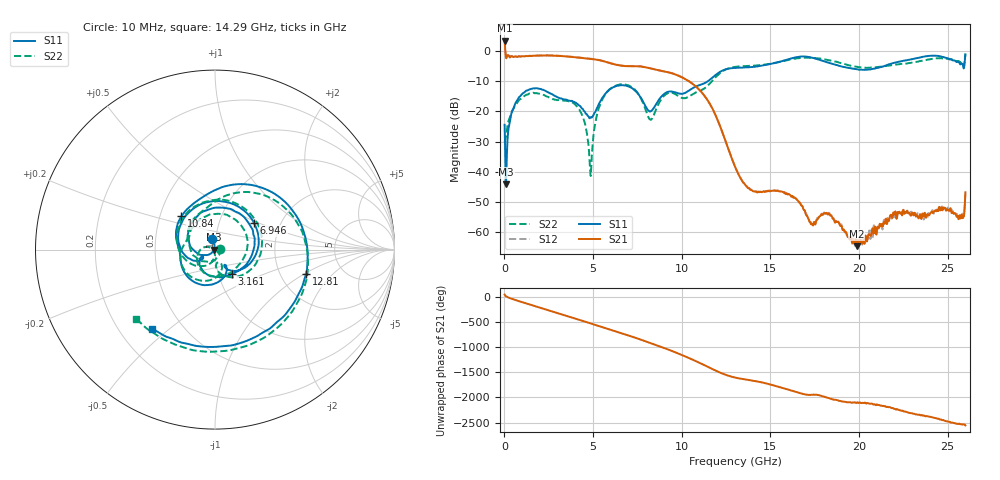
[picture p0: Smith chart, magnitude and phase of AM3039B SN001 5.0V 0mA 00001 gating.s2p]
!Agilent Technologies,E8364B,MY43040894,A.07.50.67
!Agilent E8364B: A.07.50.67
!Date: Tuesday, June 28, 2016 08:03:35
!Correction: S11(Full 2 Port(1,2))
!S21(Full 2 Port(1,2))
!S12(Full 2 Port(1,2))
!S22(Full 2 Port(1,2))
!S2P File: Measurements: S11, S21, S12, S22:
# Hz S  dB  R 50
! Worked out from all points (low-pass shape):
!   1601 points, 10 MHz to 26 GHz, reference 50 ohm
!   highest |S21| = 3.53 dB at 10 MHz (marker M1); lowest = -64.8 dB at 19.88 GHz (marker M2)
!   |S21| within 3 dB of the highest: start of sweep to 44.86 MHz
!   lowest |S11| = -44.2 dB at 91.22 MHz (marker M3), VSWR 1.01, Z = 49.4 + j0.00893 ohm
!   |S11| at or under -10 dB: start of sweep to 11.46 GHz
!   |S22| runs from -41.4 to -0.7 dB; largest |S21 - S12| = 0.024
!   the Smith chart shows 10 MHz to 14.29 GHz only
!   S11 on the Smith chart (normalised r, x): 10 MHz: 0.96, +0.11; 3.161 GHz: 1.16, -0.32; 6.946 GHz: 1.46, +0.47; 10.84 GHz: 0.64, +0.26; 12.81 GHz: 2.78, -1.03; 14.29 GHz: 0.34, -0.44
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1e7  -24.43 104.9  3.53 40.5  3.59 41.3  -30.33 10.6
9.121875e7  -44.21 179.2  -2.20 4.6  -2.10 4.6  -28.23 -60.6
7.572125e8  -16.00 158.6  -1.76 -84.1  -1.71 -83.8  -16.80 171.7
1.650619e9  -12.32 66.5  -1.50 179.4  -1.45 179.6  -13.79 70.0
3.161288e9  -15.71 -55.8  -1.57 15.8  -1.52 16.1  -16.23 -57.9
4.347081e9  -18.87 -139.3  -2.20 -115.1  -2.17 -114.9  -20.74 -170.8
4.866881e9  -21.90 -147.7  -2.53 -173.6  -2.46 -173.5  -41.43 -139.6
5.614094e9  -14.65 -177.1  -3.33 100.3  -3.28 100.4  -15.02 -163.6
6.946081e9  -11.58 34.6  -4.95 -46.6  -4.90 -46.4  -11.24 24.7
8.684162e9  -16.37 -67.7  -6.34 101.3  -6.28 101.6  -17.63 -77.0
1.084458e10  -11.58 135.2  -11.96 150.8  -11.91 150.8  -13.56 123.0
1.281008e10  -5.60 -14.8  -35.37 -150.0  -35.32 -150.0  -5.38 -21.3
1.3005e10  -5.54 -30.9  -38.36 -167.2  -38.31 -167.3  -5.18 -38.3
1.428826e10  -4.99 -128.7  -46.88 113.6  -46.60 112.8  -4.65 -139.0
1.615629e10  -2.42 83.9  -48.09 -63.6  -47.80 -62.5  -2.70 80.2
1.734208e10  -2.13 -28.5  -57.30 -149.6  -57.42 -149.8  -2.18 -20.0
1.987611e10  -5.99 130.7  -64.75 52.4  -63.27 55.0  -5.21 140.3
2.167916e10  -4.35 11.8  -56.40 -34.8  -55.89 -37.7  -4.76 16.7
2.307612e10  -2.51 -92.9  -54.53 -165.3  -53.89 -167.0  -3.72 -83.9
2.416446e10  -1.44 178.9  -53.74 118.3  -53.02 114.9  -2.47 -167.0
2.513908e10  -2.61 95.5  -52.28 29.2  -52.74 29.5  -2.65 111.2
2.6e10  -1.16 -25.7  -46.85 -38.4  -47.06 -40.2  -0.72 1.1
